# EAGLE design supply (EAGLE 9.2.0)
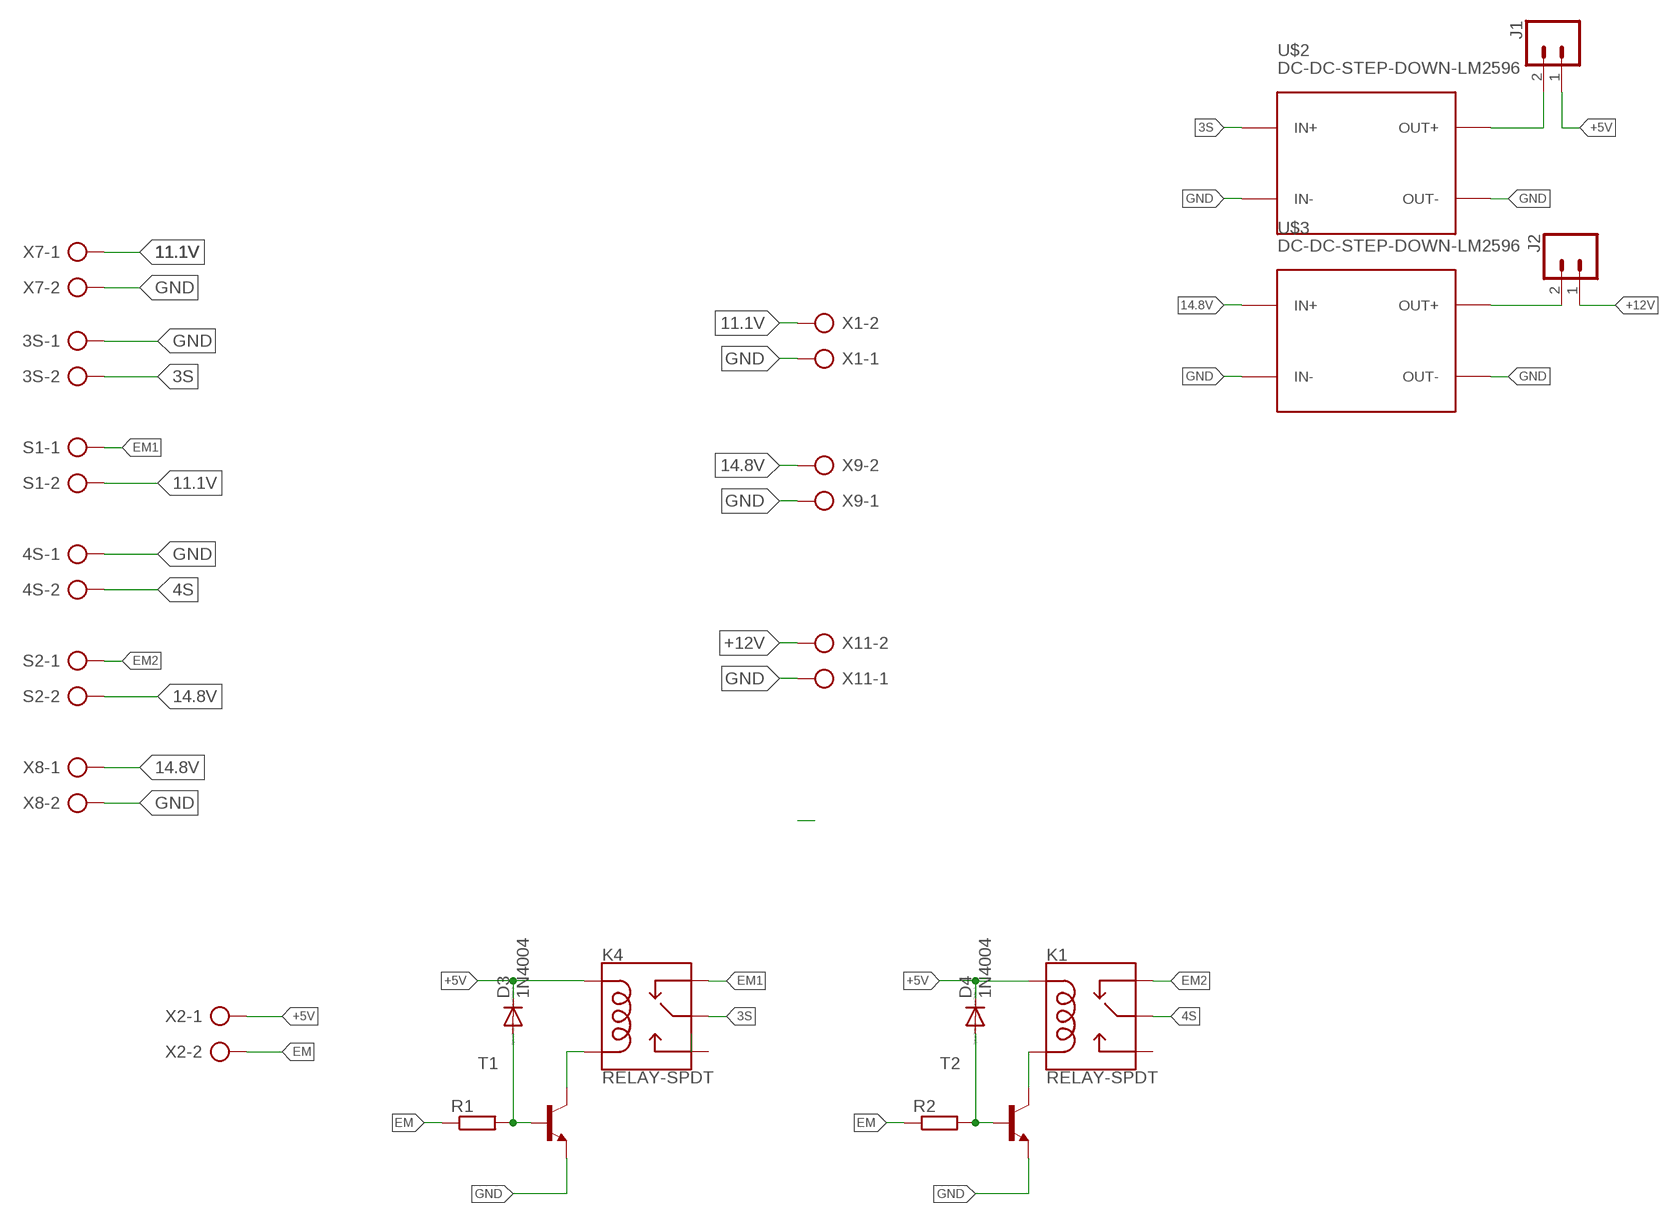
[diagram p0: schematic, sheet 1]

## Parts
3S  AK300/2  [AK300/2]
4S  AK300/2  [AK300/2]
D3  1N4004  [DO41-10]
D4  1N4004  [DO41-10]
J1  CONN_02PTH3  [1X02_LONGPADS]
J2  CONN_02PTH3  [1X02_LONGPADS]
K1  RELAY-SPDT  [RELAY_G5LE]
K4  RELAY-SPDT  [RELAY_G5LE]
R1  R-EU_0207/10  [0207/10]
R2  R-EU_0207/10  [0207/10]
S1  AK300/2  [AK300/2]
S2  AK300/2  [AK300/2]
T1  BC547B-NPN-TO92-CBE  [TO92-CBE]
T2  BC547B-NPN-TO92-CBE  [TO92-CBE]
U$2  DC-DC-STEP-DOWN-LM2596  [DC-DC-STEP-DOWN-LM2596]
U$3  DC-DC-STEP-DOWN-LM2596  [DC-DC-STEP-DOWN-LM2596]
X1  AK300/2  [AK300/2]
X2  AK300/2  [AK300/2]
X7  AK300/2  [AK300/2]
X8  AK300/2  [AK300/2]
X9  AK300/2  [AK300/2]
X11  AK300/2  [AK300/2]

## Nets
3S: 3S.2 K4.1(MAIN) U$2.IN+
4S: 4S.2 K1.1(MAIN)
11.1V: S1.2 X1.2 X7.1
14.8V: S2.2 U$3.IN+ X8.1 X9.2
+5V: D3.C D4.C J1.1 K1.2(COIL1) K4.2(COIL1) X2.1
+12V: J2.1 X11.2
EM: R1.1 R2.1 X2.2
EM1: K4.4(NC) S1.1
EM2: K1.4(NC) S2.1
GND: 3S.1 4S.1 T1.E T2.E U$2.IN- U$2.OUT- U$3.IN- U$3.OUT- X1.1 X7.2 X8.2 X9.1 X11.1
N$7: J1.2 U$2.OUT+
N$9: K1.5(COIL2) T2.C
N$10: K4.5(COIL2) T1.C
N$11: D3.A R1.2 T1.B
N$13: D4.A R2.2 T2.B
N$16: J2.2 U$3.OUT+
Unconnected: K1.3(NO) K4.3(NO)

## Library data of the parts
3S 4S S1 S2 X1 X2 X7-X9 X11 = con-ptr500:AK300/2: CONNECTOR; OC_FARNELL: unknown; OC_NEWARK: unknown
D3 D4 = diode:1N4004: DIODE
J1 J2 = SparkFun-Connectors:CONN_02: Multi connection point. Often used as Generic Header-pin footprint for 0.1 inch spaced/style header connections
K1 K4 = SparkFun-Electromechanical:RELAY-SPDT: SPDT Electromechanical Relay Single-pole, double-throw sealed relays. When current is applied to the coil, it throws a simple changeover switch, terminating the connection from the NC contact to ground and closing the NO contact. Use them to switch high voltage/high current devices. SparkFun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; PROD_ID: COMP-14214
R1 R2 = rcl:R-EU_: RESISTOR, European symbol; SPICEPREFIX: R
T1 T2 = transistor:*-NPN-: NPN Transistror BF959 corrected 2008.03.06
U$2 U$3 = diy-modules:DC-DC-STEP-DOWN-LM2596: DC/DC Step-Down Regulator based on LM2596-ADJ chip LM2596 datasheet available here: http://www.ti.com/lit/ds/symlink/lm2596.pdf Click here to find device on ebay.com

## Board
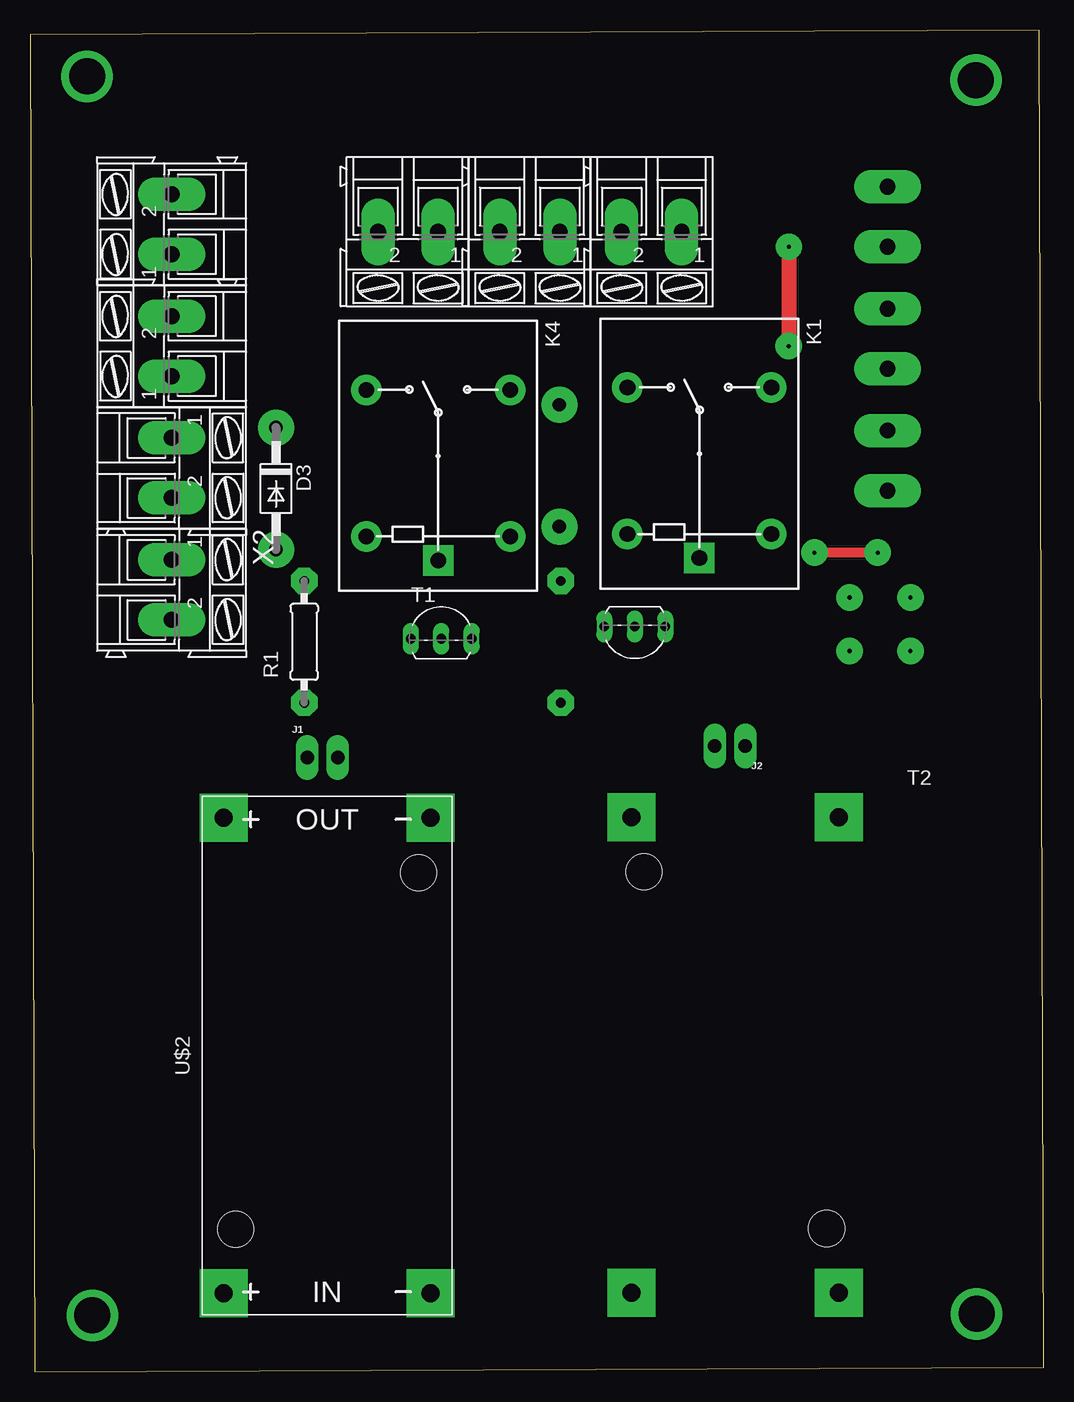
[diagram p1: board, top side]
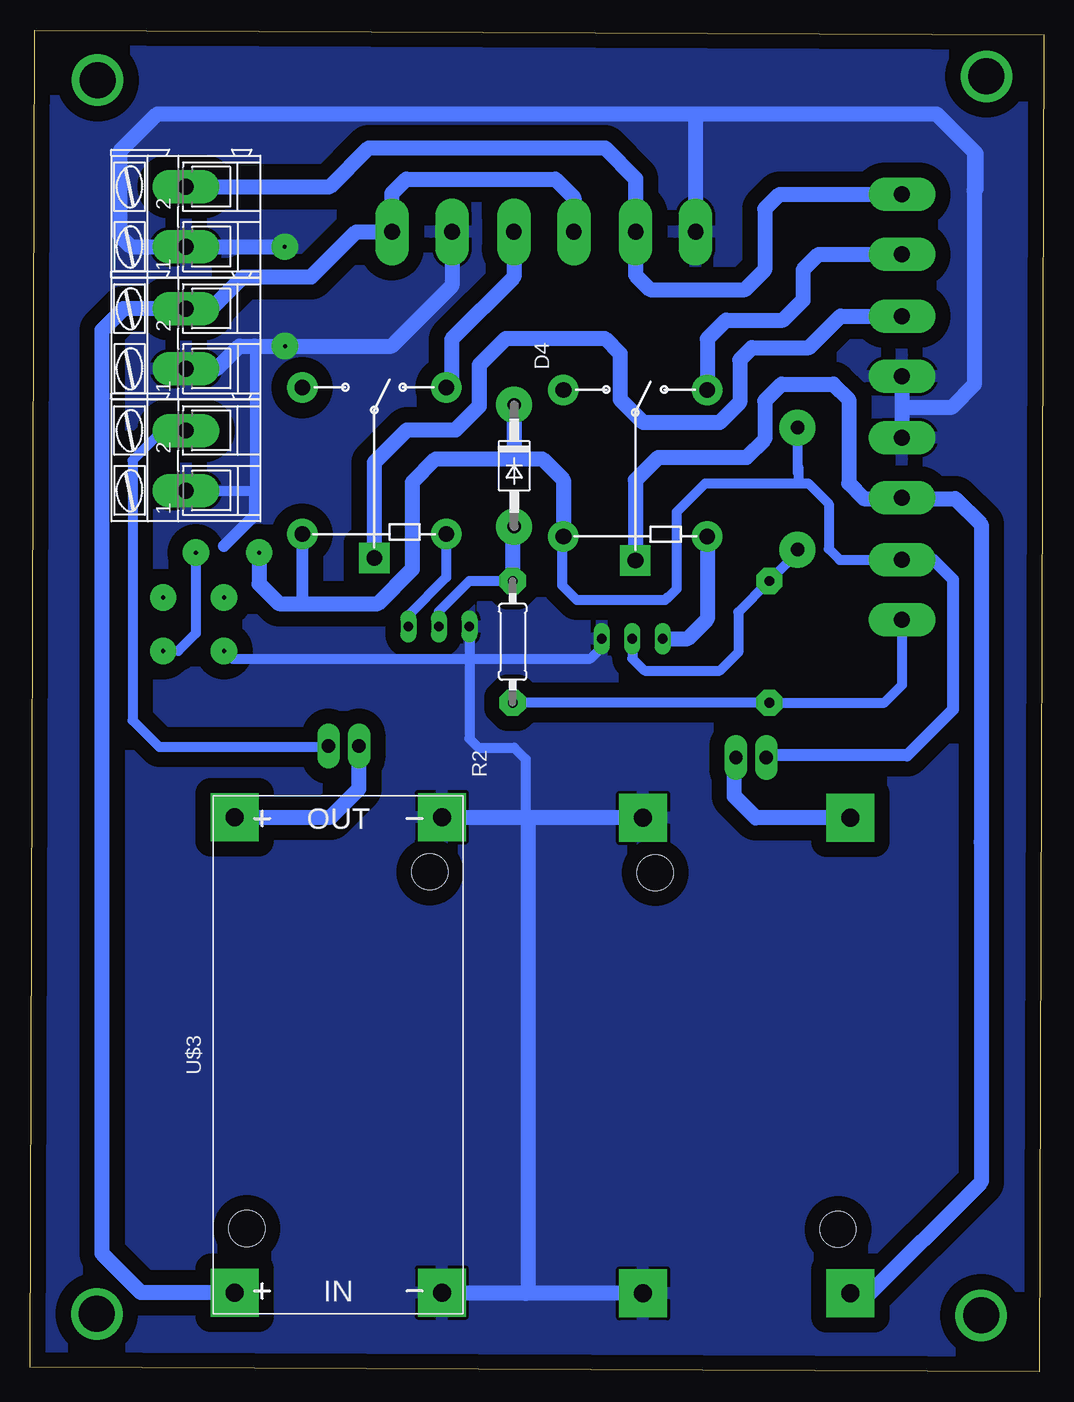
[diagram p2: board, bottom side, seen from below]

Size 84.51 x 111.81 mm. Coordinates in mm from the lower left corner, seen from the top.
Outline: 0.38,0 84.51,0.38 84.13,111.81 0,111.43 0.38,0
Copper layers (1*16): Top 0.035mm / dielectric 1.5mm / Bottom 0.035mm
Design rules "default": minimum track width 6mil, minimum drill 0.35mm, track to track 6mil, track to pad 6mil, pad to pad 6mil, via to via 6mil, smd to smd 6mil, copper to edge 40mil, drill to drill 6mil, minimum pad ring 10mil, minimum via ring 8mil, stop-mask expansion 4mil, vias tented up to drill 0mil, thermal gap 10mil

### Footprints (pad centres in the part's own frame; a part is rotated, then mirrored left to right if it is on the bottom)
AK300/2 = drill 1.321 pad 2.8 long: 1 -2.515,0; 2 2.489,0
DO41-10 = drill 1.118 pad 3: A 5.08,0; C -5.08,0
1X02_LONGPADS = drill 1.118 pad 1.88 long: 1 0,0; 2 2.54,0
RELAY_G5LE = drill 1.3 pad 2.54 square: 1 8.52,-0.005 | drill 1.3 pad 2.54: 2 6.52,5.995; 3 -5.68,5.995; 4 -5.68,-6.005; 5 6.52,-6.005
0207/10 = drill 0.8 pad 2.2 octagon: 1 -5.08,0; 2 5.08,0
TO92-CBE = drill 0.813 long: B 0,0; C -2.54,0; E 2.54,0
DC-DC-STEP-DOWN-LM2596 = drill 1.5 pad 4 square: IN+ -19.812,8.636; IN- -19.812,-8.636; OUT+ 19.812,8.636; OUT- 19.812,-8.636 | hole 3: -14.478,7.62; 15.24,-7.62

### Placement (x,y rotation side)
3S  11.81,75.31 270 top
4S  11.81,85.47 90 top
D3  20.51,73.6 270 top
D4  44.13,75.5 270 bottom
J1  23.11,51.18 0 top
J2  59.63,52.13 180 top
K1  55.82,76.33 270 top
K4  34.04,76.14 270 top
R1  22.86,60.83 90 top
R2  44.26,60.83 90 bottom
S1  11.81,95.63 90 top
S2  41.66,95 180 top
T1  34.29,61.09 0 top
T2  50.42,62.1 180 top
U$2  24.76,26.35 90 top
U$3  58.8,26.42 90 bottom
X1  71.5,96.27 90 bottom
X2  11.81,65.15 270 top
X7  31.5,95 180 top
X8  51.82,95 180 top
X9  71.5,86.11 90 bottom
X11  71.5,75.95 90 bottom

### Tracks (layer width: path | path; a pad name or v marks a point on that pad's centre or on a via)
3S
  Bottom 0.813: 3S.2 11.76,72.77 | 5.21,44.34 5.21,44.13 | 17.15,6.16 16.51,6.16 | 16.51,6.16 16.45,6.16 | 16.51,6.16 U$2.IN+
  Bottom 1.27: K4.1 34.03,74.3 32.13,76.2 24.76,76.2 23.24,77.72 23.24,80.9 21.84,82.3 17.53,82.3 16.26,81.03 16.26,74.04 14.99,72.77 11.76,72.77 7.37,72.77 5.21,70.61 5.21,44.13 5.21,15.81 14.86,6.16 16.45,6.16
4S
  Bottom 1.27: 4S.2 16.94,87.96 19.56,85.34 24.32,85.34 25.34,84.33 25.34,80.77 26.99,79.12 33.4,79.12 35.31,81.03 35.31,84.84 36.58,86.11 44.83,86.11 47.05,83.88 47.05,80.45 49.02,78.49 53.09,78.49 55.81,75.76 K1.1
11.1V
  Bottom 1.27: S1.2 22.02,98.12 23.24,96.9 23.24,91.82 24.89,90.17 32.8,90.17 34.01,91.38 X7.1 34.01,99.43 36.56,101.98 56.26,101.98 59.49,98.76 X1.2
14.8V
  Bottom 0.813: 69.34,88.65 71.45,88.65 X9.2
  Bottom 1.27: S2.2 39.17,97.84 40.7,99.38 53.15,99.38 54.36,98.17 54.36,94.97 X8.1 57.32,95 61.06,91.25 66.74,91.25 69.34,88.65 | X9.2 76.7,88.6 78.49,86.8 78.49,9.84 75.25,6.6 U$3.IN+
+5V  (via drill 0.35 pad 2.2)
  Top 0.813: v70.68,68.26 v65.41,68.26
  Bottom 0.813: 11.79,67.69 X2.1 16.99,67.67 17.91,68.58 17.91,72.33 19.62,74.04 20.45,74.04 | 72.14,60.07 70.68,61.53 v70.68,68.26 | D3.C 20.51,75.5 | 20.51,75.5 20.51,74.93 | K4.2 40.13,69.52 40.13,65.53 38.93,64.33 31.56,64.33 31.37,64.52 31.31,64.52 30.61,65.21 30.61,71.63 28.19,74.04 20.45,74.04 | 20.51,75.5 20.45,75.44 20.45,74.04
  Bottom 1.016: X2.1 9.18,67.67 7.56,66.04 7.56,55.18 11.37,51.37 22.92,51.37 J1.1 | 50.67,76.07 44.13,76.07 | 61.91,64.01 55.5,64.01 | 63.75,64.01 61.91,64.01 | K1.2 61.81,64.11 61.91,64.01
  Bottom 1.27: 44.13,76.07 D4.C 44.13,79.37 | K4.2 40.03,74.32 41.78,76.07 50.67,76.07 52.64,74.1 52.64,66.87 55.5,64.01 63.75,64.01 65.41,65.66 v65.41,68.26
+12V
  Bottom 0.813: X11.2 71.55,78.49 73.41,78.49 75.95,75.95 75.95,54.29 73.72,52.07 59.69,52.07 J2.1
EM
  Bottom 0.813: X2.2 11.81,57.21 13.27,55.75 R1.1 R2.1
EM1
  Bottom 1.27: S1.1 18.77,93.12 20.07,91.82 20.07,89.28 21.72,87.63 26.48,87.63 28.03,86.08 K4.4
EM2
  Bottom 1.27: S2.1 44.17,91.21 49.36,86.03 49.36,82.46 K1.4
GND  (via drill 0.35 pad 2.2)
  Top 1.27: v63.27,93.75 63.27,85.5 v63.25,85.47
  Bottom 0.813: 67.69,59.44 47.88,59.44 | T2.E 47.88,59.44 | 65.79,85.47 65.79,73.41 65.81,73.43 X11.1 | T1.E 36.83,60.39 37.78,59.44 47.88,59.44 | 47.88,59.44 47.88,52.77 47.12,52.01 44.13,52.01 43.18,51.05 43.18,46.35 42.99,46.16
  Bottom 1.016: 5.78,98.43 5.65,98.55 | 65.79,73.41 65.79,71.37 68.33,68.83
  Bottom 1.27: 11.81,80.39 3S.1 | 4S.1 11.81,80.39 | 63.25,93.73 v63.27,93.75 X1.1 76.1,93.75 77.03,94.68 77.03,101.69 73.89,104.83 8.94,104.83 5.65,101.54 5.65,98.55 | X8.2 49.33,90.5 54.36,85.47 v63.25,85.47 65.79,85.47 67.06,85.47 68.96,83.57 71.48,83.57 X9.1 | 11.81,80.39 7.62,80.39 5.78,82.23 5.78,98.43 5.78,101.55 | 29.02,104.07 29.01,104.05 X7.2 | U$2.IN- 43.18,6.54 | 43.18,6.54 50.42,6.54 50.67,6.79 50.36,6.79 U$3.IN- | U$2.OUT- 42.99,46.16 | 42.99,46.16 50.1,46.16 U$3.OUT- | 42.99,46.16 42.99,6.73 43.18,6.54
  pour Bottom (isolate 1.27): 0.13,111.44 84.45,111.44 84.45,-0.13 0.13,-0.13
N$1  (via drill 0.35 pad 2.2)
  other vias: 73.41,64.52
N$2  (via drill 0.35 pad 2.2)
  other vias: 73.41,60.07
N$3  (via drill 3 pad 4.3)
  other vias: 4.76,107.95
N$4  (via drill 3 pad 4.3)
  other vias: 5.21,4.7
N$5  (via drill 3 pad 4.3)
  other vias: 78.93,4.83
N$6  (via drill 3 pad 4.3)
  other vias: 78.87,107.63
N$7
  Bottom 1.27: U$2.OUT+ 24,46.16 25.78,47.94 25.78,50.29 25.46,50.61 25.46,50.99 J1.2
N$9
  Bottom 0.813: K1.5 49.81,66.2 52.96,63.06 T2.C
N$10
  Bottom 1.27: K4.5 28.03,62.71 29.65,61.09 T1.C
N$11
  Bottom 0.813: D3.A 20.51,68.26 R1.2 25.46,63.31 25.46,59.94 26.99,58.42 33.27,58.42 34.29,59.44 T1.B
N$12  (via drill 0.35 pad 2.2)
  other vias: 68.33,60.07
N$13
  Bottom 0.813: 44.39,66.99 44.26,66.87 R2.2 47.88,65.91 50.42,63.37 T2.B
  Bottom 1.27: R2.2 44.26,70.29 D4.A
N$14  (via drill 0.35 pad 2.2)
  other vias: 68.33,64.52
N$16
  Bottom 1.27: U$3.OUT+ 59.44,46.23 57.09,48.58 J2.2

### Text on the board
tValues: G | 3S | 12V | SAKLAR | G | 11.1V | 4S | G | G | 14.8V | G

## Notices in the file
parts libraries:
SparkFun-Electromechanical: Licensing: Creative Commons ShareAlike 4.0 International - https://creativecommons.org/licenses/by-sa/4.0
diy-modules: Released under the Creative Commons Attribution 4.0 International License: http://creativecommons.org/licenses/by/4.0
